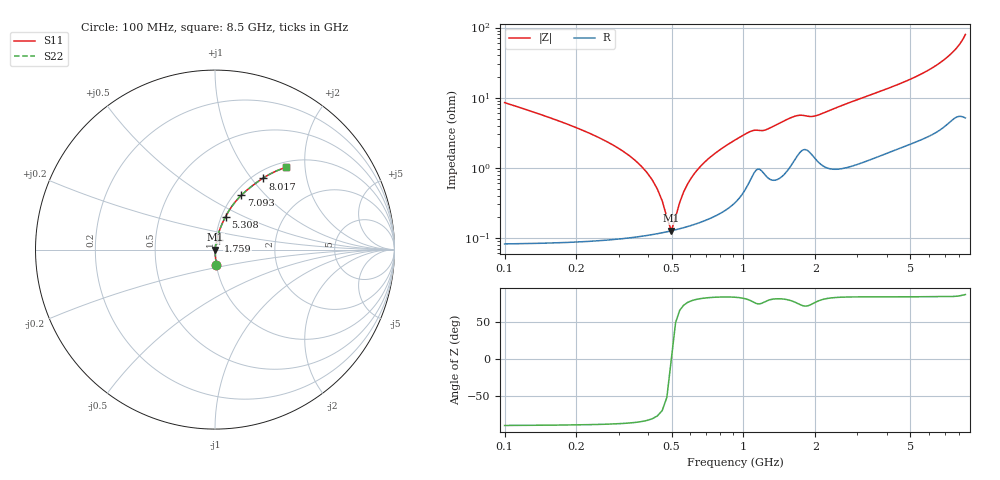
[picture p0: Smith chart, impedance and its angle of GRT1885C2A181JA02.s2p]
!Murata Part Number: GRT1885C2A181JA02
!These Parameters are Measured in Series Mode Connection
!Data Generated on Jun 19, 2026
!  o--ll--o
!Port1  Port2
!  o------o
!Operation Temp=25[degC], DC Bias Voltage=0[V]
!Freq. Start=100[MHz] Stop=9[GHz] 401[Steps]
# Hz S RI R 50
!Freq.(Hz) S11(Real) S11(Imag) S21(Real) S21(Imag) S12(Real) S12(Imag) S22(Real) S22(Imag)
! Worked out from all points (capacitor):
!   401 points, 100 MHz to 8.5 GHz, reference 50 ohm
!   read as one part in series: C = 180 pF near 142 MHz
!   lowest |Z| = 126 mohm at 499 MHz (marker M1)
!   series resonance near 499 MHz, so ESL is about 570 pH
!   S11 on the Smith chart (normalised r, x): 100 MHz: 1.00, -0.17; 1.759 GHz: 1.04, +0.11; 5.308 GHz: 1.05, +0.40; 7.093 GHz: 1.08, +0.74; 8.017 GHz: 1.11, +1.14; 8.5 GHz: 1.10, +1.59
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1e8  0.00796 -0.0842  0.992 0.0842  0.992 0.0842  0.00796 -0.0842
3.52e8  0.00118 -0.0127  0.9988 0.0127  0.9988 0.0127  0.00118 -0.0127
4.15e8  0.00115 -0.0066  0.9988 0.0066  0.9988 0.0066  0.00115 -0.0066
4.57e8  0.00119 -0.00314  0.9988 0.00314  0.9988 0.00314  0.00119 -0.00314
4.99e8  0.00126 6e-07  0.9987 -6e-07  0.9987 -6e-07  0.00126 6e-07
5.41e8  0.00135 0.0029  0.9986 -0.0029  0.9986 -0.0029  0.00135 0.0029
5.83e8  0.00147 0.00561  0.9985 -0.00561  0.9985 -0.00561  0.00147 0.00561
6.25e8  0.00162 0.00818  0.9984 -0.00818  0.9984 -0.00818  0.00162 0.00818
6.88e8  0.00189 0.0118  0.9981 -0.0118  0.9981 -0.0118  0.00189 0.0118
7.93e8  0.0025 0.0176  0.9975 -0.0176  0.9975 -0.0176  0.0025 0.0176
1.066e9  0.00752 0.0317  0.9925 -0.0317  0.9925 -0.0317  0.00752 0.0317
1.507e9  0.0107 0.0464  0.9893 -0.0464  0.9893 -0.0464  0.0107 0.0464
1.759e9  0.02 0.0513  0.98 -0.0513  0.98 -0.0513  0.02 0.0513
1.99e9  0.0161 0.0513  0.9839 -0.0513  0.9839 -0.0513  0.0161 0.0513
2.914e9  0.0184 0.087  0.9816 -0.087  0.9816 -0.087  0.0184 0.087
4.3e9  0.0374 0.1387  0.9626 -0.1387  0.9626 -0.1387  0.0374 0.1387
5.308e9  0.0589 0.1839  0.9411 -0.1839  0.9411 -0.1839  0.0589 0.1839
5.707e9  0.0707 0.2052  0.9293 -0.2052  0.9293 -0.2052  0.0707 0.2052
7.093e9  0.1469 0.303  0.8531 -0.303  0.8531 -0.303  0.1469 0.303
7.114e9  0.1488 0.3048  0.8512 -0.3048  0.8512 -0.3048  0.1488 0.3048
8.017e9  0.2649 0.3963  0.7351 -0.3963  0.7351 -0.3963  0.2649 0.3963
8.5e9  0.3951 0.4577  0.6049 -0.4577  0.6049 -0.4577  0.3951 0.4577
